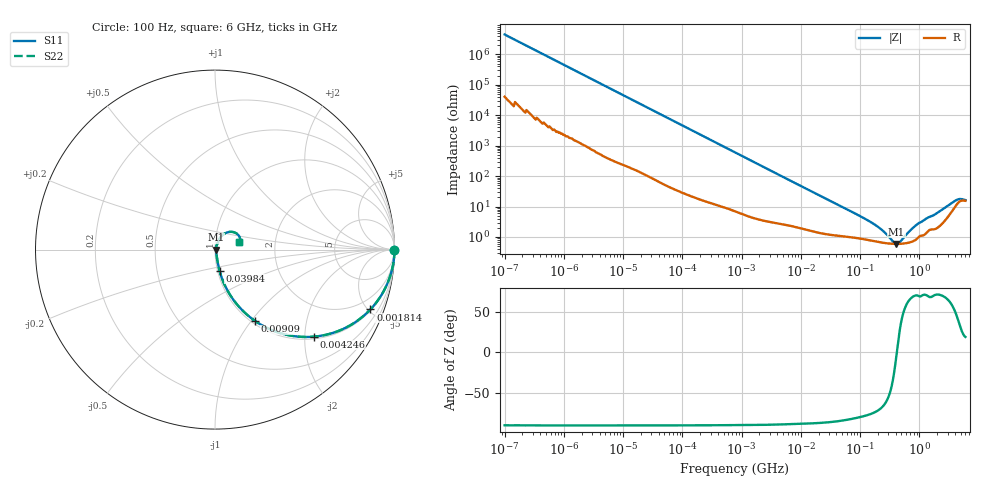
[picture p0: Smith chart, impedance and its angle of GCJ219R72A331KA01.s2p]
!Murata Part Number: GCJ219R72A331KA01
!These Parameters are Measured in Series Mode Connection
!Data Generated on Mar 13, 2026
!  o--ll--o
!Port1  Port2
!  o------o
!Operation Temp=25[degC], DC Bias Voltage=0[V]
!Freq. Start=100[Hz] Stop=6[GHz] 401[Steps]
# Hz S RI R 50
!Freq.(Hz) S11(Real) S11(Imag) S21(Real) S21(Imag) S12(Real) S12(Imag) S22(Real) S22(Imag)
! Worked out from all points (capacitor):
!   401 points, 100 Hz to 6 GHz, reference 50 ohm
!   read as one part in series: C = 353 pF near 109 Hz
!   lowest |Z| = 597 mohm at 408.7 MHz (marker M1)
!   series resonance near 417 MHz, so ESL is about 410 pH
!   S11 on the Smith chart (normalised r, x): 100 Hz: open; 1.814 MHz: 1.08, -5.16; 4.246 MHz: 1.06, -2.22; 9.09 MHz: 1.04, -1.05; 39.84 MHz: 1.02, -0.24; 6 GHz: 1.31, +0.11
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100  1 -2.22e-05  2e-07 2.22e-05  2e-07 2.22e-05  1 -2.22e-05
458  1 -0.000101  6e-07 0.000101  6e-07 0.000101  1 -0.000101
2008  1 -0.000441  2.4e-06 0.000441  2.4e-06 0.000441  1 -0.000441
40335  0.9999 -0.00877  0.000126 0.00877  0.000126 0.00877  0.9999 -0.00877
241822  0.9969 -0.0521  0.00313 0.0521  0.00313 0.0521  0.9969 -0.0521
774597  0.9713 -0.1613  0.0287 0.1613  0.0287 0.1613  0.9713 -0.1613
1813585  0.8657 -0.3335  0.1343 0.3335  0.1343 0.3335  0.8657 -0.3335
4246196  0.5503 -0.4851  0.4497 0.4851  0.4497 0.4851  0.5503 -0.4851
9090158  0.2243 -0.3983  0.7757 0.3983  0.7757 0.3983  0.2243 -0.3983
1.555665e7  0.0985 -0.2742  0.9015 0.2742  0.9015 0.2742  0.0985 -0.2742
3.983537e7  0.0252 -0.1173  0.9748 0.1173  0.9748 0.1173  0.0252 -0.1173
1.596157e8  0.00827 -0.0277  0.9917 0.0277  0.9917 0.0277  0.00827 -0.0277
2.283698e8  0.00685 -0.0163  0.9932 0.0163  0.9932 0.0163  0.00685 -0.0163
3.124326e8  0.00613 -0.00762  0.9939 0.00762  0.9939 0.00762  0.00613 -0.00762
4.087225e8  0.00591 -0.000523  0.9941 0.000523  0.9941 0.000523  0.00591 -0.000523
4.674818e8  0.00595 0.00305  0.9941 -0.00305  0.9941 -0.00305  0.00595 0.00305
8.749838e8  0.00864 0.0224  0.9914 -0.0224  0.9914 -0.0224  0.00864 0.0224
1.309207e9  0.0146 0.0371  0.9854 -0.0371  0.9854 -0.0371  0.0146 0.0371
2.562649e9  0.0353 0.0747  0.9647 -0.0747  0.9647 -0.0747  0.0353 0.0747
4.009986e9  0.1004 0.098  0.8996 -0.098  0.8996 -0.098  0.1004 0.098
4.796499e9  0.1345 0.0751  0.8655 -0.0751  0.8655 -0.0751  0.1345 0.0751
6e9  0.1358 0.0403  0.8642 -0.0403  0.8642 -0.0403  0.1358 0.0403
